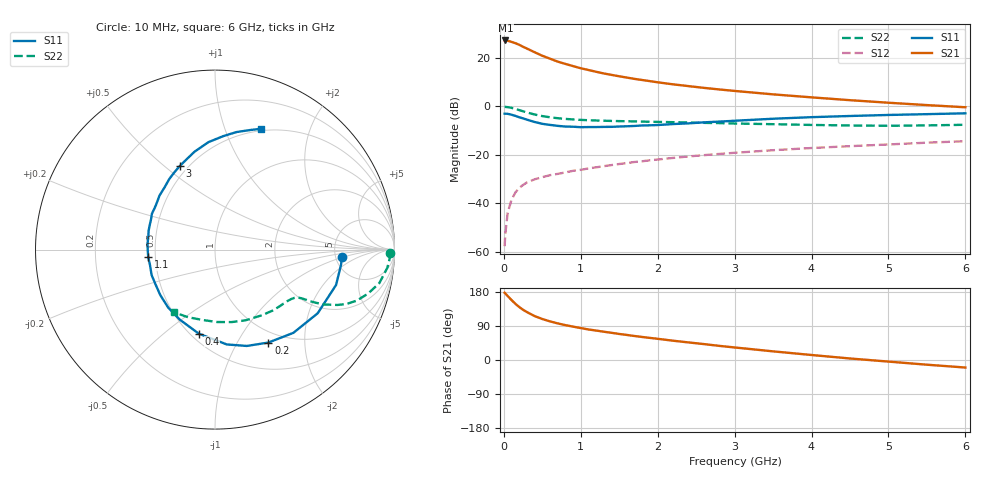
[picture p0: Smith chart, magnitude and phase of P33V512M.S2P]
! SIEMENS Small Signal Semiconductors
! BFP181
! Si NPN RF Bipolar Junction Transistor in SOT143
! VCE = 3.5 V  IC = 12 mA
! Common Emitter S-Parameters:  March  1996
# GHz  S  MA  R  50
!  f  S11  S21  S12  S22
! GHz  MAG  ANG  MAG  ANG  MAG  ANG  MAG  ANG
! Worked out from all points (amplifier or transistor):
!   36 points, 10 MHz to 6 GHz, reference 50 ohm
!   highest |S21| = 27.2 dB at 20 MHz (marker M1)
!   |S21| within 3 dB of that: start of sweep to 276.8 MHz
!   unconditionally stable (mu >= 1): 982.5 MHz to 5.997 GHz
!   at 250 MHz: K = 0.38, MSG = 28.5 dB, |S12| = -32.4 dB
!   at 1.4 GHz: K = 1.12, MAG = 16.5 dB, |S12| = -24.2 dB
!   at 6 GHz: K = 1.00, MSG = 7.0 dB, |S12| = -14.4 dB
!   S11 on the Smith chart (normalised r, x): 10 MHz: 5.67, -0.92; 200 MHz: 0.84, -1.36; 400 MHz: 0.55, -0.67; 1.1 GHz: 0.46, -0.05; 3 GHz: 0.45, +0.56; 6 GHz: 0.48, +1.34
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0.01  0.707 -3.3  22.93 177.4  0.0013 76.8  0.9747 -1.0
0.02  0.7075 -6.8  23.01 175.5  0.0024 73.7  0.9771 -2.2
0.05  0.7027 -16.3  22.72 168.7  0.0064 85.8  0.9656 -6.0
0.1  0.6732 -31.8  21.48 158.2  0.0118 73.8  0.9346 -11.5
0.15  0.6371 -46.7  20.21 148.3  0.0167 68.3  0.8878 -16.0
0.2  0.5973 -60.1  18.72 139.9  0.0207 63.8  0.8394 -19.8
0.25  0.5654 -71.7  17.04 132.5  0.0239 60.8  0.7924 -22.5
0.3  0.5326 -82.9  15.67 126.5  0.0269 57.7  0.7494 -24.3
0.4  0.477 -100.9  13.14 115.9  0.0312 53.5  0.6807 -26.7
0.5  0.437 -116.5  11.11 108.2  0.0346 51.4  0.6309 -27.9
0.6  0.4151 -128.9  9.675 101.9  0.038 50.5  0.5963 -28.6
0.7  0.3965 -140.2  8.417 96.6  0.0404 50.5  0.5707 -29.0
0.9  0.3806 -158.2  6.796 88.1  0.0468 50.3  0.538 -29.9
1.1  0.3746 -173.4  5.647 80.6  0.0524 50.8  0.5185 -31.2
1.3  0.3775 175.0  4.788 74.6  0.0583 50.9  0.5061 -33.0
1.6  0.3888 159.0  3.935 66.1  0.0675 50.5  0.4934 -36.0
2.2  0.4317 135.7  2.857 50.9  0.0863 48.2  0.4723 -44.1
3  0.5054 112.9  2.088 33.1  0.1102 43.2  0.4433 -57.1
3.5  0.5564 102.0  1.773 22.8  0.1246 39.9  0.4293 -66.6
4.5  0.6341 85.8  1.344 4.0  0.151 31.8  0.4036 -88.5
5.5  0.6918 74.1  1.065 -12.4  0.1783 24.6  0.4055 -111.6
6  0.7203 69.2  0.96 -19.9  0.1913 20.5  0.4176 -123.3
